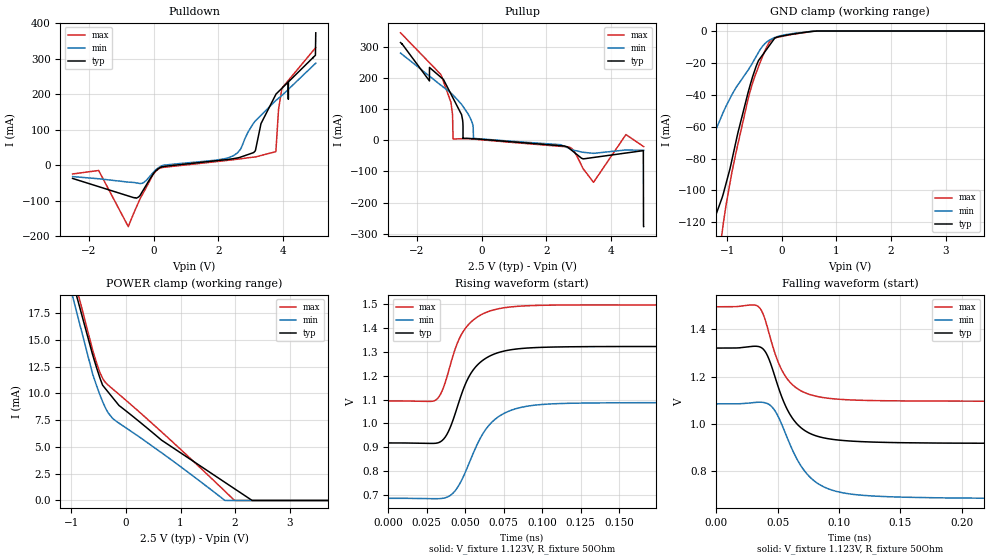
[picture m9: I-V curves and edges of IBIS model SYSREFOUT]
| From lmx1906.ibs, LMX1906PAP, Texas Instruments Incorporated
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|   Model SYSREFOUT
[Model]   SYSREFOUT
Model_type   Output
Polarity   Non-Inverting
Vmeas = 1.25
Vref = 1.25
Cref = 2pF
Rref = 50
|   typ   min   max
C_comp   0.4pF   0.38pF   0.424pF
[Voltage Range]   2.5   2.4   2.6
[Temperature Range]   27   105   -40
[Pullup Reference]   2.5   2.4   2.6
[Pulldown Reference]   0   0   0
[Power Clamp Reference]   2.5   2.4   2.6
[GND Clamp Reference]   0   0   0
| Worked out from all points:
|   slope of the pulldown table from 0 to 0.375 V, typ, clamps not added: 18.6 ohm
|   slope of the pullup table from 0 to 0.375 V, typ, clamps not added: 118 ohm
|   falling waveform, V_fixture 1.123V, R_fixture 50Ohm: 20-80 % time 20.9ps typ, 25.9ps min, 19.2ps max; typ from 1.32 V to 0.917 V
|   rising waveform, V_fixture 1.123V, R_fixture 50Ohm: 20-80 % time 16ps typ, 19.4ps min, 15ps max; typ from 0.917 V to 1.32 V
[Pulldown]
|   Voltage   I(typ)   I(min)   I(max)
-2.5V     -37.33mA   -32.12mA   -24.72mA
-1.698V   -60.39mA   -38.23mA   -14.9mA
-782.5mV  -86.7mA    -47.66mA   -173mA
192.5mV   -7.251mA   -4.395mA   -8.193mA
2.45V     18.22mA    26.24mA    15.44mA
3.083V    35.53mA    118.4mA    22.68mA
3.763V    198.3mA    181.8mA    37.89mA
3.958V    216.9mA    196.5mA    217.3mA
4.154V    185.9mA    213.7mA    238.8mA
4.154V    234.5mA    213.7mA    238.8mA
4.99V     309.8mA    286.7mA    330.5mA
5V        373mA      287.6mA    331.6mA
[GND Clamp]
|   Voltage   I(typ)   I(min)   I(max)
-2.5V     -242.9mA   -160.5mA   -404.5mA
-1.863V   -183.1mA   -116.5mA   -326.5mA
-1.363V   -130mA     -75.86mA   -200.4mA
-1.225V   -117mA     -63.34mA   -161mA
-1.091V   -104.4mA   -52.46mA   -125.9mA
-917.5mV  -81.5mA    -40.18mA   -89.25mA
-610mV    -37.66mA   -24.18mA   -41.6mA
-427.6mV  -18.59mA   -13.47mA   -22.48mA
-280mV    -11.6mA    -7.003mA   -10.25mA
-167.5mV  -6.277mA   -4.663mA   -5.032mA
652.6mV   0A         0A         0A
5V        0A         0A         0A
[Pullup]
|   Voltage   I(typ)   I(min)   I(max)
-2.5V     314mA      280.2mA    345.3mA
-1.248V   201.8mA    176.4mA    209.4mA
-940mV    147.6mA    151.6mA    118.7mA
-880mV    135.5mA    145.7mA    4.182mA
-572.6mV  6.103mA    108.9mA    5.026mA
-250mV    4.974mA    6.324mA    3.771mA
2.728V    -27.88mA   -27.67mA   -22.78mA
3.455V    -55.2mA    -41.93mA   -134.7mA
4.452V    -40.91mA   -31.05mA   18.37mA
4.99V     -33.22mA   -32.26mA   -19.63mA
4.995V    -276.8mA   -32.27mA   -19.99mA
5V        -277.3mA   -32.28mA   -20.35mA
[POWER Clamp]
|   Voltage   I(typ)   I(min)   I(max)
-2.5V     61.82mA    57.18mA    62.44mA
-1.607V   32.32mA    31.52mA    33.74mA
-616.6mV  13.73mA    11.94mA    14.18mA
-490mV    11.66mA    10.05mA    12.14mA
-427.6mV  10.77mA    9.241mA    11.43mA
-250mV    9.65mA     7.706mA    10.45mA
-127.8mV  8.881mA    7.226mA    9.92mA
652.6mV   5.637mA    4.458mA    6.405mA
1.812V    1.697mA    5.925uA    869uA
1.985V    1.111mA    0A         22.4uA
2.312V    0A         0A         0A
5V        0A         0A         0A
[Ramp]
R_load = 50
|   typ   min   max
dV/dt_r   0.242291/1.60314e-11   0.240554/1.94423e-11   0.240809/1.50268e-11
dV/dt_f   0.242291/2.09104e-11   0.240554/2.58812e-11   0.240809/1.91718e-11
[Falling Waveform]
V_fixture = 1.123V
V_fixture_min = 0.887V
V_fixture_max = 1.3V
R_fixture = 50Ohm
C_fixture = 0F
|   Time   V(typ)   V(min)   V(max)
0s        1.321V     1.085V     1.496V
33ps      1.329V     1.092V     1.5V
38ps      1.318V     1.091V     1.467V
43ps      1.274V     1.083V     1.384V
53ps      1.12V      1.003V     1.232V
66ps      999.2mV    849.6mV    1.15V
81ps      950.6mV    755mV      1.118V
103ps     930.6mV    709.5mV    1.104V
240ps     918.5mV    685.9mV    1.096V
1.25ns    917.3mV    684.4mV    1.094V
[Rising Waveform]
V_fixture = 1.123V
V_fixture_min = 0.887V
V_fixture_max = 1.3V
R_fixture = 50Ohm
C_fixture = 0F
|   Time   V(typ)   V(min)   V(max)
0s        917.3mV    684.4mV    1.094V
30ps      915.6mV    682.8mV    1.095V
35ps      927.6mV    684.1mV    1.137V
40ps      978.8mV    695.3mV    1.238V
47ps      1.111V     752.3mV    1.367V
52ps      1.191V     823.8mV    1.414V
58ps      1.246V     914.2mV    1.448V
70ps      1.294V     1.02V      1.48V
89ps      1.316V     1.07V      1.494V
1.25ns    1.321V     1.085V     1.496V
